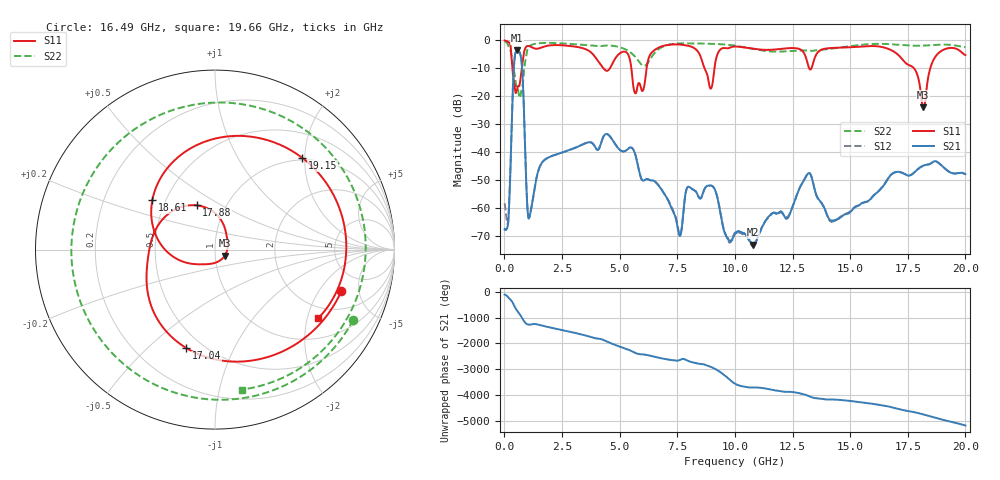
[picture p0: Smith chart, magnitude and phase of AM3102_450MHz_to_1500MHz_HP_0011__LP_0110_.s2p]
!Agilent Technologies,E8364B,MY43040894,A.07.50.67
!Agilent E8364B: A.07.50.67
!Date: Thursday, January 11, 2018 05:31:38
!Correction: S11(Full 2 Port(1,2))
!S21(Full 2 Port(1,2))
!S12(Full 2 Port(1,2))
!S22(Full 2 Port(1,2))
!S2P File: Measurements: S11, S21, S12, S22:
# Hz S  dB  R 50
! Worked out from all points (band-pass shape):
!   1601 points, 10 MHz to 20 GHz, reference 50 ohm
!   highest |S21| = -3.56 dB at 559.7 MHz (marker M1); lowest = -73.0 dB at 10.77 GHz (marker M2)
!   |S21| within 3 dB of the highest: 441.7 MHz to 728.9 MHz (287.2 MHz wide, 49.1 % of centre)
!   lowest |S11| = -23.8 dB at 18.18 GHz (marker M3), VSWR 1.14, Z = 55.6 - j3.76 ohm
!   |S11| at or under -10 dB: 5.509 GHz to 6.17 GHz (660.5 MHz wide, 11.3 % of centre); 8.684 GHz to 9.111 GHz (427.5 MHz wide, 4.81 % of centre); 17.77 GHz to 18.47 GHz (702.5 MHz wide, 3.88 % of centre)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
!   |S22| runs from -20.5 to -0.4 dB; largest |S21 - S12| = 0.0026
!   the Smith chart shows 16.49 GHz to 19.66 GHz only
!   S11 on the Smith chart (normalised r, x): 16.49 GHz: 3.22, -3.28; 17.04 GHz: 0.41, -0.67; 17.88 GHz: 0.73, +0.39; 18.61 GHz: 0.42, +0.29; 19.15 GHz: 0.96, +1.95; 19.66 GHz: 1.61, -2.35
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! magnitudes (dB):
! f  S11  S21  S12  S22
! 10 MHz  0.0  -67.5  -58.2  -0.4
! 172.4 MHz  -0.6  -64.7  -63.6  -2.1
! 559.7 MHz  -17.3  -3.6  -3.6  -17.4
! 747.1 MHz  -10.4  -7.7  -7.7  -17.8
! 1.084 GHz  -2.1  -63.2  -62.9  -2.2
! 3.346 GHz  -2.7  -37.3  -37.3  -1.6
! 5.682 GHz  -18.9  -40.9  -40.9  -5.9
! 6.682 GHz  -2.6  -51.8  -51.6  -3.2
! 8.956 GHz  -17.2  -51.8  -51.8  -1.2
! 10.01 GHz  -2.2  -69.1  -68.8  -1.9
! 10.77 GHz  -3.0  -73.0  -73.2  -3.0
! 13.34 GHz  -9.6  -49.2  -49.2  -3.8
! 14.23 GHz  -2.7  -64.5  -64.7  -2.9
! 16.49 GHz  -2.6  -51.4  -51.3  -1.3
! 16.68 GHz  -3.1  -48.9  -48.9  -1.3
! 17.04 GHz  -4.9  -47.0  -47.0  -1.6
! 17.88 GHz  -11.5  -46.4  -46.4  -1.9
! 18.18 GHz  -23.8  -44.7  -44.8  -1.9
! 18.61 GHz  -7.0  -43.3  -43.3  -1.7
! 19.15 GHz  -3.0  -46.0  -46.1  -1.5
! 19.66 GHz  -3.2  -47.5  -47.4  -2.0
! 20 GHz  -5.3  -47.8  -47.8  -2.4
